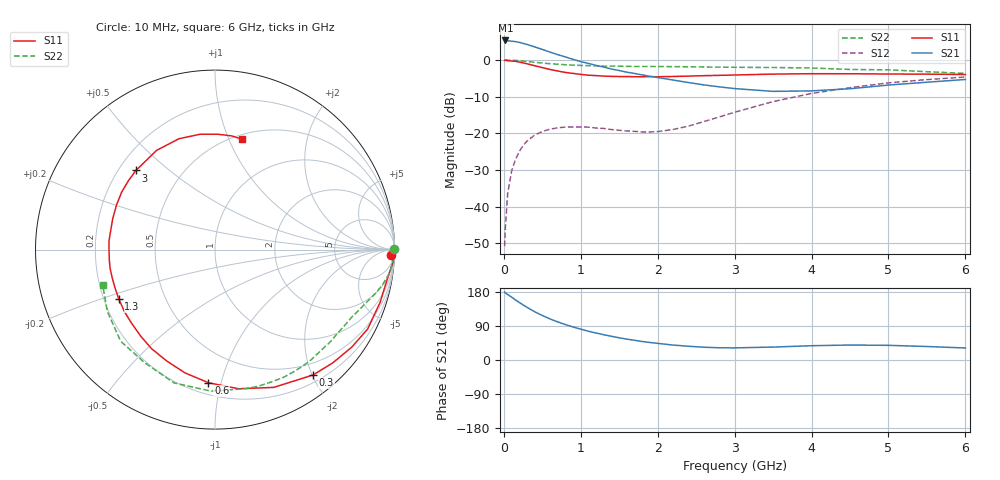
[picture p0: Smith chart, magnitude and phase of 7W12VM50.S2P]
! Infineon Technologies  Discrete & RF Semiconductors
! BFS17W
! Si NPN RF Bipolar Junction Transistor in SOT323
! VCE = 12 V  IC = 0.5 mA
! Common Emitter S-Parameters:  August  1999
# GHz  S  MA  R  50
!  f  S11  S21  S12  S22
! GHz  MAG  ANG  MAG  ANG  MAG  ANG  MAG  ANG
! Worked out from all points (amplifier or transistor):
!   36 points, 10 MHz to 6 GHz, reference 50 ohm
!   highest |S21| = 5.3 dB at 20 MHz (marker M1)
!   |S21| within 3 dB of that: start of sweep to 576.5 MHz
!   unconditionally stable (mu >= 1): 1.268 GHz to end of sweep
!   at 250 MHz: K = 0.21, MSG = 13.9 dB, |S12| = -23.4 dB
!   at 1.4 GHz: K = 1.12, MAG = 6.2 dB, |S12| = -19.0 dB
!   at 6 GHz: K = 1.08, MAG = -2.0 dB, |S12| = -4.6 dB
!   S11 on the Smith chart (normalised r, x): 10 MHz: 30, -49; 300 MHz: 0.31, -2.02; 600 MHz: 0.28, -0.91; 1.3 GHz: 0.26, -0.23; 3 GHz: 0.27, +0.39; 6 GHz: 0.55, +1.12
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0.01  0.982 -1.7  1.827 179.3  0.0029 79.2  0.9999 0.1
0.02  0.9945 -3.9  1.843 177.2  0.0053 93.0  0.9985 -0.8
0.05  0.9754 -9.1  1.826 172.8  0.0151 86.8  0.9968 -2.2
0.1  0.9657 -17.8  1.801 166.0  0.0302 79.4  0.9916 -4.3
0.15  0.9587 -27.5  1.778 158.7  0.0438 73.3  0.9849 -6.4
0.2  0.9358 -35.5  1.737 151.9  0.0564 70.3  0.9759 -8.4
0.3  0.8872 -51.9  1.629 139.1  0.0783 60.4  0.9534 -11.9
0.4  0.8346 -66.9  1.507 127.5  0.0945 52.5  0.9296 -14.9
0.5  0.7863 -80.4  1.392 117.5  0.106 46.3  0.9074 -17.5
0.6  0.7427 -92.8  1.279 108.4  0.114 41.2  0.8884 -19.9
0.8  0.6762 -113.5  1.099 93.5  0.1217 34.0  0.8608 -24.3
1.1  0.6196 -138.8  0.896 75.8  0.1212 28.8  0.8365 -30.5
1.3  0.6025 -152.8  0.799 66.7  0.1165 28.8  0.8255 -35.0
1.7  0.5914 -174.6  0.654 52.0  0.1064 35.9  0.8148 -44.2
2.2  0.5951 163.3  0.532 39.4  0.1127 56.3  0.8104 -56.5
3  0.6233 135.0  0.407 32.0  0.1938 74.5  0.7937 -77.5
3.5  0.6415 120.5  0.373 34.1  0.2708 73.4  0.7888 -91.6
4  0.6494 108.1  0.379 37.7  0.3498 67.7  0.7771 -107.0
4.5  0.6483 97.3  0.405 39.5  0.4183 60.5  0.7418 -121.9
5  0.6432 88.8  0.455 38.7  0.4877 53.0  0.7327 -135.8
5.5  0.6403 81.6  0.497 35.6  0.5398 45.4  0.6918 -150.1
6  0.6329 76.0  0.542 31.7  0.5858 38.4  0.6558 -162.7
